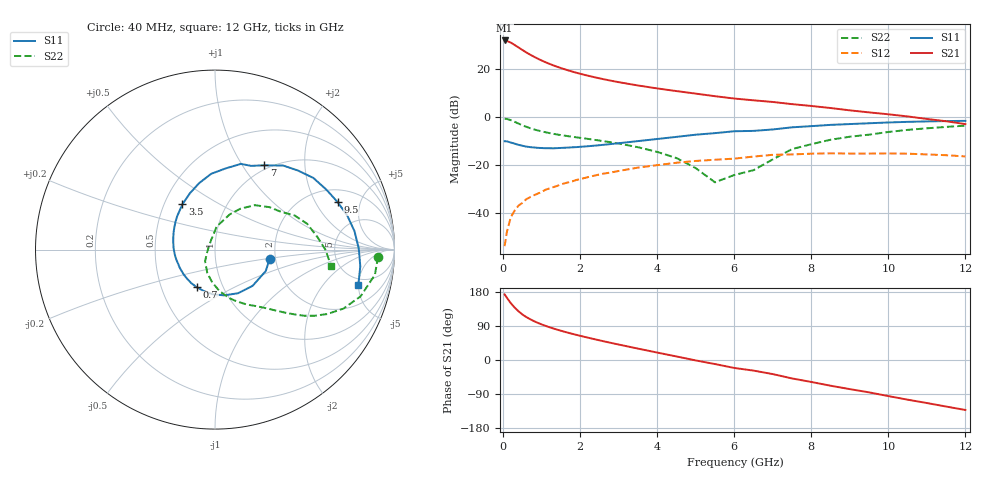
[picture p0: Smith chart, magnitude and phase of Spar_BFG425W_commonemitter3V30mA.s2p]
! Filename: 330bfg425.001
! BFG425W Field C1
! V1=8.550E-001V,V2=3.000E+000V, I1=4.198E-004A, I2=3.001E-002A
# GHz  S  MA  R 50
!  S11  S21  S12  S22
!Freq(GHz)  Mag  Ang  Mag  Ang  Mag  Ang  Mag  Ang
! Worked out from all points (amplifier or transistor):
!   44 points, 40 MHz to 12 GHz, reference 50 ohm
!   highest |S21| = 31.8 dB at 40 MHz (marker M1)
!   |S21| within 3 dB of that: start of sweep to 408 MHz
!   unconditionally stable (mu >= 1): start of sweep to 44.53 MHz; 1.114 GHz to end of sweep
!   at 700 MHz: K = 0.85, MSG = 29.8 dB, |S12| = -33.6 dB
!   at 2.4 GHz: K = 1.17, MAG = 17.9 dB, |S12| = -24.4 dB
!   at 12 GHz: K = 1.35, MAG = 3.2 dB, |S12| = -16.5 dB
!   S11 on the Smith chart (normalised r, x): 40 MHz: 1.86, -0.21; 700 MHz: 0.75, -0.34; 3.5 GHz: 0.62, +0.35; 7 GHz: 0.94, +1.26; 9.5 GHz: 2.73, +3.11; 12 GHz: 4.13, -4.96
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0.04  0.309 -9.4  39.11 173.2  0.002 81.2  0.909 -2.5
0.1  0.307 -22.9  38.18 164.1  0.004 80.7  0.902 -8.9
0.2  0.291 -43.9  35.26 150.0  0.008 74.6  0.852 -17.8
0.3  0.275 -62.1  31.52 138.4  0.011 70.9  0.787 -24.7
0.4  0.26 -78.7  27.96 128.6  0.014 68.7  0.722 -29.8
0.5  0.249 -93.2  24.8 120.3  0.016 66.6  0.666 -33.6
0.6  0.239 -105.3  22.1 113.5  0.019 65.3  0.619 -36.5
0.7  0.233 -115.5  19.84 107.8  0.021 64.1  0.579 -38.8
0.9  0.225 -133.1  16.33 98.1  0.025 62.8  0.519 -42.4
1.2  0.221 -153.2  12.75 86.6  0.032 60.7  0.458 -46.8
1.6  0.226 -173.8  9.79 74.4  0.041 57.8  0.404 -52.1
2.2  0.243 163.0  7.203 59.0  0.055 51.7  0.346 -61.1
2.8  0.27 144.3  5.66 45.2  0.069 44.5  0.294 -70.9
3.5  0.311 125.7  4.502 30.1  0.087 34.9  0.232 -83.8
4.5  0.381 103.4  3.438 9.4  0.11 19.9  0.138 -108.1
5.5  0.456 82.6  2.689 -10.7  0.127 4.2  0.043 -168.6
6.5  0.508 66.7  2.207 -28.0  0.148 -8.3  0.077 98.4
7  0.544 59.7  2.038 -37.2  0.161 -16.0  0.129 85.9
8.5  0.678 36.1  1.523 -67.9  0.173 -45.2  0.332 48.2
9.5  0.733 21.1  1.235 -85.4  0.171 -61.8  0.424 29.7
10.5  0.784 7.5  1.018 -104.7  0.17 -80.2  0.533 15.7
12  0.822 -13.7  0.704 -131.9  0.149 -109.8  0.654 -8.1
